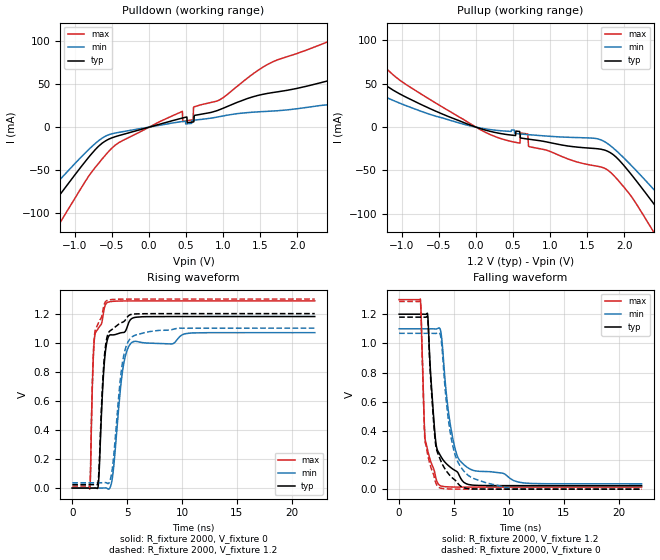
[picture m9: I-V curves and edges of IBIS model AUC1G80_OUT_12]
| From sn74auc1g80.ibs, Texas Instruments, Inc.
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[Model]   AUC1G80_OUT_12
Model_type  Output
Vref =   0
Rref =   2000
Cref =   15p
Vmeas =   0.6
| variable   typ   min   max
C_comp   6.57pF   2.68pF   16.98pF
| C_pullup   6.11pF   2.68pF   16.98pF
| C_pulldown   7.03pF   5.28pF   15.32pF
[Temperature Range]   40   100   -40
| Ambient temperature   25   85   -40
[Voltage range]   1.2   1.1   1.3
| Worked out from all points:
|   slope of the pulldown table from 0 to 0.18 V, typ, clamps not added: 41.7 ohm
|   slope of the pullup table from 0 to 0.18 V, typ, clamps not added: 39.2 ohm
|   rising waveform, R_fixture 2000, V_fixture 0: 20-80 % time 513ps typ, 832ps min, 321ps max; typ from 0 V to 1.18 V
|   falling waveform, R_fixture 2000, V_fixture 1.2: 20-80 % time 796ps typ, 1.17ns min, 530ps max; typ from 1.2 V to 0.024 V
|   rising waveform, R_fixture 2000, V_fixture 1.2: 20-80 % time 502ps typ, 818ps min, 314ps max; typ from 0.024 V to 1.2 V
|   falling waveform, R_fixture 2000, V_fixture 0: 20-80 % time 834ps typ, 1.18ns min, 497ps max; typ from 1.18 V to 0 V
[Pulldown]
| AUC1G80_OUT_12
|   Voltage   I(typ)   I(min)   I(max)
-3.6V     -353mA     -295.2mA   -432.4mA
-1.74V    -139.9mA   -112.1mA   -184.4mA
-1.205V   -78.45mA   -61mA      -111.1mA
-405mV    -9.738mA   -5.991mA   -17.81mA
450mV     10.56mA    6.521mA    18.26mA
455mV     10.67mA    6.577mA    6.451mA
590mV     5.951mA    7.923mA    8.587mA
605mV     6.428mA    8.061mA    23.39mA
1.605V    39.16mA    18.35mA    72.9mA
2.9V      63.71mA    22.49mA    116.1mA
3.425V    52.26mA    23.6mA     133.9mA
7.2V      67.12mA    31.57mA    126.6mA
[Pullup]
| AUC1G80_OUT_12
|   Voltage   I(typ)   I(min)   I(max)
-3.6V     224.8mA    101.7mA    291.7mA
-2.7V     158.7mA    66.33mA    205.2mA
-2.18V    115.9mA    79.99mA    155.4mA
-1.825V   88.42mA    63.34mA    122mA
65mV      -1.832mA   -1.08mA    -3.199mA
700mV     -13.77mA   -8.609mA   -7.935mA
715mV     -13.95mA   -8.713mA   -22.38mA
1.78V     -27.93mA   -19.17mA   -49.63mA
2.41V     -89.51mA   -72.81mA   -122.6mA
2.7V      -122.8mA   -100.4mA   -163.2mA
3.05V     -163.5mA   -134.4mA   -211.9mA
7.2V      -644.6mA   -548.6mA   -776.4mA
[Ramp]
| AUC1G80_OUT_12
| variable   typ   min   max
dV/dt_r   0.71/5.14E-10   0.65/8.37E-10   0.78/3.22E-10
dV/dt_f   0.71/7.92E-10   0.64/1.17E-09   0.77/5.29E-10
R_load = 2000
[Rising Waveform]
| AUC1G80_OUT_12
R_fixture =   2000
C_fixture =   0
L_fixture =   0
V_fixture =   0
V_fixture_min = 0
V_fixture_max = 0
|   Time   V(typ)   V(min)   V(max)
0s        6.8nV      28.92nV    711.7pV
1.59ns    -2.598uV   -1.09uV    -7.218mV
1.955ns   57.22uV    -4.945uV   956.5mV
2.35ns    7.74mV     2.45uV     1.096V
2.815ns   742.5mV    541.8uV    1.191V
3.13ns    995.4mV    -326.4uV   1.273V
3.67ns    1.053V     78.25mV    1.284V
4.67ns    1.07V      846.8mV    1.287V
5.43ns    1.167V     1.002V     1.287V
22.1ns    1.18V      1.069V     1.287V
[Falling Waveform]
| AUC1G80_OUT_12
R_fixture =   2000
C_fixture =   0
L_fixture =   0
V_fixture =   1.2
V_fixture_min = 1.1
V_fixture_max = 1.3
|   Time   V(typ)   V(min)   V(max)
0s        1.2V       1.1V       1.3V
1.935ns   1.2V       1.1V       1.304V
2.32ns    1.2V       1.1V       402.2mV
2.575ns   1.207V     1.1V       275mV
3.24ns    401.2mV    1.099V     116mV
3.665ns   243.5mV    1.106V     28mV
4.865ns   139.2mV    357.9mV    14.78mV
6.12ns    37.03mV    154.4mV    14.05mV
11.41ns   24.12mV    42.18mV    13.9mV
22.1ns    24.02mV    36.67mV    13.88mV
[Rising Waveform]
| AUC1G80_OUT_12
R_fixture =   2000
C_fixture =   0
L_fixture =   0
V_fixture =   1.2
V_fixture_min = 1.1
V_fixture_max = 1.3
|   Time   V(typ)   V(min)   V(max)
0s        23.98mV    36.63mV    13.86mV
1.59ns    23.97mV    36.63mV    6.945mV
1.945ns   24.01mV    36.63mV    964.6mV
2.325ns   28.76mV    36.64mV    1.126V
2.805ns   772.6mV    37.09mV    1.226V
3.1ns     1.013V     36.81mV    1.287V
3.635ns   1.092V     124.1mV    1.297V
4.62ns    1.142V     883.6mV    1.3V
5.445ns   1.195V     1.04V      1.3V
22.1ns    1.2V       1.1V       1.3V
[Falling Waveform]
| AUC1G80_OUT_12
R_fixture =   2000
C_fixture =   0
L_fixture =   0
V_fixture =   0
V_fixture_min = 0
V_fixture_max = 0
|   Time   V(typ)   V(min)   V(max)
0s        1.18V      1.069V     1.287V
1.935ns   1.18V      1.069V     1.291V
2.355ns   1.179V     1.069V     330.6mV
2.6ns     1.173V     1.069V     238.6mV
3.18ns    424.1mV    1.068V     90.15mV
3.585ns   234.7mV    1.073V     14.14mV
3.835ns   187.6mV    1.022V     6.288mV
4.84ns    77.85mV    314.2mV    837.8uV
6.285ns   4.109mV    95.23mV    157.7uV
22.1ns    41.69uV    20.26uV    14.94uV
